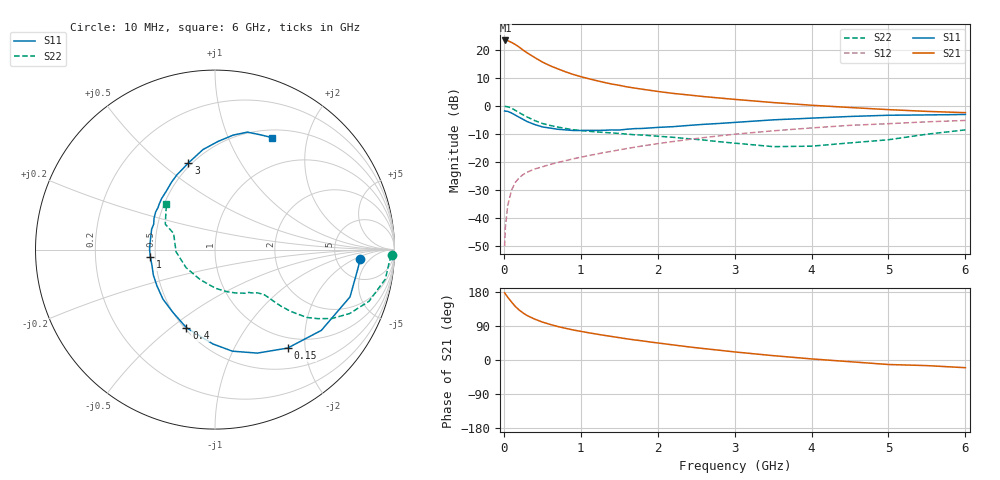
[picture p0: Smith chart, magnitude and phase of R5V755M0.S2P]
! SIEMENS Small Signal Semiconductors
! BFR183
! Si NPN RF Bipolar Junction Transistor in SOT23
! VCE = 0.75 V  IC = 5 mA
! Common Emitter S-Parameters:  May  1996
# GHz  S  MA  R  50
!  f  S11  S21  S12  S22
! GHz  MAG  ANG  MAG  ANG  MAG  ANG  MAG  ANG
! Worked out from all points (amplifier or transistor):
!   36 points, 10 MHz to 6 GHz, reference 50 ohm
!   highest |S21| = 23.4 dB at 20 MHz (marker M1)
!   |S21| within 3 dB of that: start of sweep to 229.1 MHz
!   unconditionally stable (mu >= 1): 950.5 MHz to 3.029 GHz
!   at 250 MHz: K = 0.43, MSG = 22.3 dB, |S12| = -24.6 dB
!   at 1.4 GHz: K = 1.09, MAG = 10.2 dB, |S12| = -16.3 dB
!   at 6 GHz: K = 0.95, MSG = 1.4 dB, |S12| = -5.2 dB
!   S11 on the Smith chart (normalised r, x): 10 MHz: 8.65, -2.78; 150 MHz: 0.82, -1.67; 400 MHz: 0.51, -0.57; 1 GHz: 0.47, -0.04; 3 GHz: 0.48, +0.62; 6 GHz: 0.60, +1.47
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0.01  0.8105 -3.9  14.66 177.4  0.0031 90.8  0.9855 -1.9
0.02  0.8025 -7.9  14.75 174.2  0.0067 86.6  0.9741 -3.9
0.05  0.7971 -19.3  14.65 165.9  0.0164 80.2  0.9632 -9.8
0.1  0.7441 -37.2  13.61 153.1  0.0312 71.8  0.9054 -18.5
0.15  0.6817 -53.6  12.46 141.0  0.0429 64.8  0.8305 -25.4
0.2  0.6233 -67.7  11.2 131.8  0.0518 59.9  0.7563 -30.5
0.25  0.5742 -80.3  9.928 124.2  0.059 56.2  0.6898 -33.9
0.3  0.5257 -91.3  8.915 117.6  0.0649 54.0  0.6352 -36.5
0.4  0.4636 -110.1  7.32 108.0  0.0742 51.9  0.5452 -39.2
0.5  0.4205 -124.1  6.072 100.2  0.0814 51.1  0.4846 -40.6
0.6  0.4004 -136.4  5.22 94.0  0.0894 51.0  0.4467 -41.2
0.7  0.3816 -147.7  4.591 88.4  0.097 51.5  0.4184 -41.6
0.8  0.372 -157.3  4.064 83.7  0.1045 51.9  0.3942 -42.0
1  0.3625 -173.5  3.324 75.6  0.1206 53.2  0.3623 -43.0
1.1  0.3645 179.9  3.061 72.0  0.1288 53.3  0.3519 -44.2
1.6  0.3818 152.8  2.183 55.8  0.1725 53.1  0.3123 -50.4
2.2  0.4244 129.6  1.669 39.8  0.2302 50.2  0.2739 -62.4
3  0.5054 107.0  1.305 21.3  0.311 42.4  0.2154 -89.3
3.5  0.5617 96.8  1.145 11.5  0.3575 36.3  0.1865 -116.3
4.5  0.6457 81.0  0.934 -4.5  0.4481 23.5  0.2175 -177.0
5.5  0.6879 68.4  0.796 -14.8  0.5181 11.6  0.3112 152.9
6  0.7007 62.8  0.755 -20.3  0.5482 3.7  0.3719 136.7
